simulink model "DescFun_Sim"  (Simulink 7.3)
settings: Solver=ode3  StartTime=0.0  StopTime=500  FixedStep=0.002  RelTol=1e-3
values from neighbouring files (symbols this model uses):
  E = EE(j)    [DF_Calculate.m]    (also in run_fcs.m = eye(n))
  omg = 0.05    [DF_Calculate.m]
undefined symbols (not defined in the file or in its folder): Coulomb_Damper

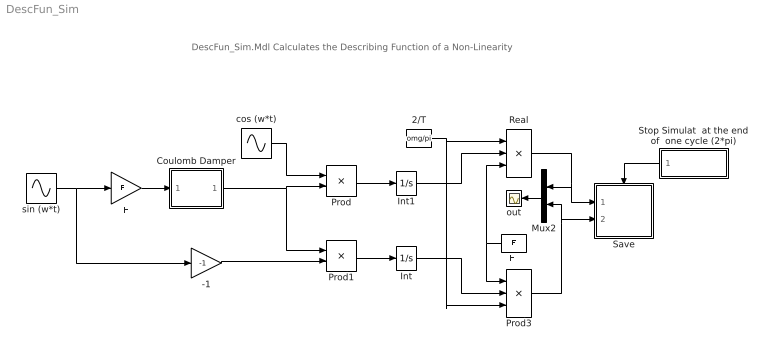
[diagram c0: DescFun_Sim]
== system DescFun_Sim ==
  note: DescFun_Sim.Mdl Calculates the Describing Function of a Non-Linearity
  -1 : Gain  Gain=-1  ParameterDataType=sfix(16)  ParameterScaling=2^0  OutDataType=sfix(16)  OutScaling=2^0
  2/T : Constant  Value=omg/pi  OutDataType=sfix(16)  OutScaling=2^0
  Coulomb Damper : Subsystem
  E : Gain  Gain=E  ParameterDataType=sfix(16)  ParameterScaling=2^0  OutDataType=sfix(16)  OutScaling=2^0
  "E " : Constant  Value=E  OutDataType=sfix(16)  OutScaling=2^0
  Int : Integrator
  Int1 : Integrator
  Mux2 : Mux  Inputs=2
  Prod : Product  OutDataType=sfix(16)  OutScaling=2^0
  Prod1 : Product  OutDataType=sfix(16)  OutScaling=2^0
  Prod3 : Product  Inputs=/**  OutDataType=sfix(16)  OutScaling=2^0
  Real : Product  Inputs=**/  OutDataType=sfix(16)  OutScaling=2^0
  Save : Subsystem
  Stop Simulat  at the end of  one cycle (2*pi) : Subsystem
  cos (w*t) : Sin  Amplitude=1  Bias=0  Frequency=omg  Phase=pi/2  Samples=10  SampleTime=0
  out : Scope
  sin (w*t) : Sin  Amplitude=1  Bias=0  Frequency=omg  Phase=0  Samples=10  SampleTime=0
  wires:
  sin (w*t)/1 -> -1/1, E/1
  Coulomb Damper/1(Fcd) -> Prod/2, Prod1/1
  cos (w*t)/1 -> Prod/1
  -1/1 -> Prod1/2
  E/1 -> Coulomb Damper/1(Ext)
  Prod1/1 -> Int/1
  Prod/1 -> Int1/1
  "E "/1 -> Real/3, Prod3/1
  Int1/1 -> Real/2
  Int/1 -> Prod3/2
  2/T/1 -> Real/1, Prod3/3
  Prod3/1 -> Save/2(imag), Mux2/2
  Mux2/1 -> out/1
  Real/1 -> Save/1(real), Mux2/1
  Stop Simulat  at the end of  one cycle (2*pi)/1(Triger at Stop) -> Save/Trigger

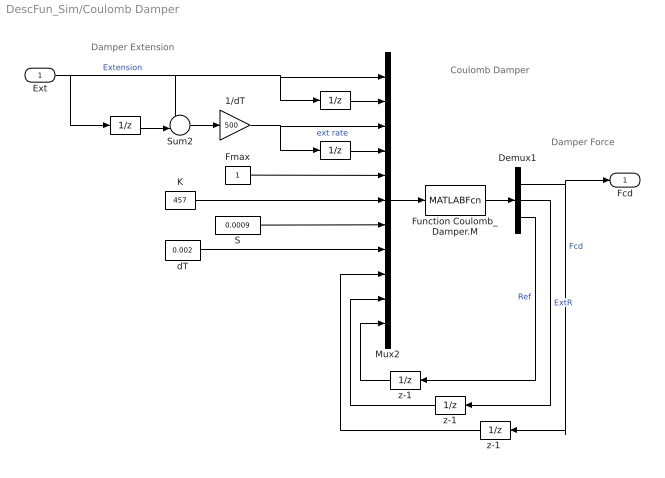
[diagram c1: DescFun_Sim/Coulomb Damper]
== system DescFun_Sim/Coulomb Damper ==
  note: Coulomb Damper
  note: Damper Force
  note: Damper Extension
  Ext : Inport  OutDataType=sfix(16)  OutScaling=2^0
  " " : UnitDelay  SampleTime=0.002
  "   " : UnitDelay  SampleTime=0.002
  "       " : UnitDelay  SampleTime=0.002
  " z-1 " : UnitDelay  SampleTime=0.002
  1/dT : Gain  Gain=500  ParameterDataType=sfix(16)  ParameterScaling=2^0  OutDataType=sfix(16)  OutScaling=2^0
  Demux1 : Demux  Outputs=3
  Fmax : Constant  OutDataType=sfix(16)  OutScaling=2^0
  Function Coulomb_Damper.M : MATLABFcn  MATLABFcn=Coulomb_Damper(u(1), u(2), u(3), u(4), u(5),u(6),u(7),u(8), u(9),u(10),u(11) )  OutputDimensions=3  SampleTime=0.002
  K : Constant  Value=457  OutDataType=sfix(16)  OutScaling=2^0
  Mux2 : Mux  Inputs=11
  S : Constant  Value=0.0009  OutDataType=sfix(16)  OutScaling=2^0
  Sum2 : Sum  Inputs=+-|  OutDataType=sfix(16)  OutScaling=2^0
  dT : Constant  Value=0.002  OutDataType=sfix(16)  OutScaling=2^0
  z-1 : UnitDelay  SampleTime=0.002
  "z-1 " : UnitDelay  SampleTime=0.002
  Fcd : Outport  OutDataType=sfix(16)  OutScaling=2^0
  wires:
  Function Coulomb_Damper.M/1 -> Demux1/1
  Demux1/3 -> z-1/1  "Ref"
  Demux1/2 -> " z-1 "/1  "ExtR"
  Demux1/1 -> "z-1 "/1, Fcd/1  "Fcd"
  z-1/1 -> Mux2/11
  " z-1 "/1 -> Mux2/10
  "z-1 "/1 -> Mux2/9
  Ext/1 -> "       "/1, Sum2/1, " "/1, Mux2/1  "Extension"
  " "/1 -> Mux2/2
  "   "/1 -> Mux2/4
  "       "/1 -> Sum2/2
  Sum2/1 -> 1/dT/1
  1/dT/1 -> "   "/1, Mux2/3  "ext rate"
  Fmax/1 -> Mux2/5
  K/1 -> Mux2/6
  S/1 -> Mux2/7
  Mux2/1 -> Function Coulomb_Damper.M/1
  dT/1 -> Mux2/8

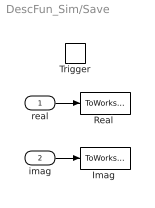
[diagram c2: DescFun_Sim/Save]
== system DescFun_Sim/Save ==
  real : Inport  OutDataType=sfix(16)  OutScaling=2^0
  imag : Inport  Port=2  OutDataType=sfix(16)  OutScaling=2^0
  Trigger : TriggerPort
  "Imag " : ToWorkspace  VariableName=DF_imag  SampleTime=-1  SaveFormat=Array
  "Real " : ToWorkspace  VariableName=DF_real  SampleTime=-1  SaveFormat=Array
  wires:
  real/1 -> "Real "/1
  imag/1 -> "Imag "/1

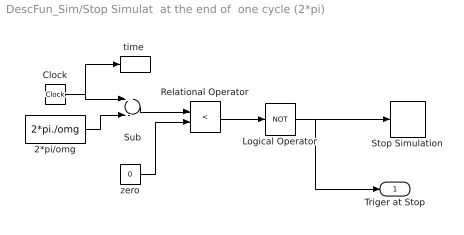
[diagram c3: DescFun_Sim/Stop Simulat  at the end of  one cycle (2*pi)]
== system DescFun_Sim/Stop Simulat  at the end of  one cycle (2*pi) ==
  2*pi/omg : Constant  Value=2*pi./omg  OutDataType=sfix(16)  OutScaling=2^0
  Clock : Clock
  Logical Operator : Logic  Operator=NOT  AllPortsSameDT=off  OutDataTypeMode=boolean  OutDataTypeStr=boolean
  Relational Operator : RelationalOperator  Operator=<  LogicOutDataTypeMode=boolean  OutDataTypeStr=boolean
  Stop Simulation : Stop
  Sub : Sum  Inputs=+-  OutDataType=sfix(16)  OutScaling=2^-10
  "time " : ToWorkspace  VariableName=time  SampleTime=-1  SaveFormat=Array
  zero : Constant  Value=0  OutDataType=sfix(16)  OutScaling=2^0
  Triger at Stop : Outport  OutDataType=sfix(16)  OutScaling=2^0
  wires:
  Clock/1 -> Sub/1, "time "/1
  2*pi/omg/1 -> Sub/2
  Sub/1 -> Relational Operator/1
  zero/1 -> Relational Operator/2
  Relational Operator/1 -> Logical Operator/1
  Logical Operator/1 -> Stop Simulation/1, Triger at Stop/1
